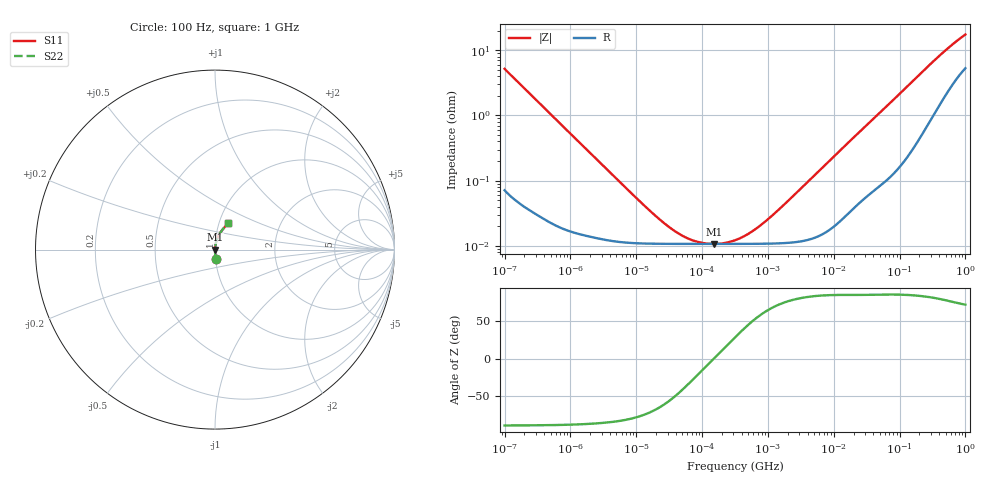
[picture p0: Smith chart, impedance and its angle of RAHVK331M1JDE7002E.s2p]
! RAHVK331M1JDE7002E  S-PARAMETER MODEL  (AEC-Q200 qualified)
! Model Generated by ELNA Corporation (http://www.ty-top.com)
! Version 1.0
! ELNA Control No.201026
! Copyright (c) 2020 ELNA CO.,LTD. All Rights Reserved.
! Products Name : CONDUCTIVE POLYMER HYBRID ALUMINUM ELECTROLYTIC CAPACITORS
! Characteristics :
!  Capacitance  :  330uF  ,  Rated voltage  :  6.3V
!  Operating Temp. Range  :  -55 to +125 degC  ,  Endurance  :  4000hr at 125 degC
!  Dimension D  :  6.3mm  ,  Dimension L  :  7.7mm
! Frequency Range : 100Hz - 1GHz
! External Node Assignments :
!  1  o---| |---o  2
# MHz S RI R 50
!Freq[MHz].  S11 Real  S11 Imag  S21 Real  S21 Imag  S12 Real  S12 Imag  S22 Real  S22 Imag
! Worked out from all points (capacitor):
!   401 points, 100 Hz to 1 GHz, reference 50 ohm
!   read as one part in series: C = 307 uF near 108 Hz
!   lowest |Z| = 10.7 mohm at 153.1 kHz (marker M1)
!   series resonance near 150.2 kHz, so ESL is about 3.7 nH
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0.0001  0.00338 -0.0515  0.9966 0.0515  0.9966 0.0515  0.00338 -0.0515
0.000113  0.00272 -0.0457  0.9973 0.0457  0.9973 0.0457  0.00272 -0.0457
0.000309  0.000582 -0.0168  0.9994 0.0168  0.9994 0.0168  0.000582 -0.0168
0.001488  0.00016 -0.00354  0.9998 0.00354  0.9998 0.00354  0.00016 -0.00354
0.009495  0.00011 -0.000559  0.9999 0.000559  0.9999 0.000559  0.00011 -0.000559
0.022131  0.000108 -0.000236  0.9999 0.000236  0.9999 0.000236  0.000108 -0.000236
0.037368  0.000107 -0.000134  0.9999 0.000134  0.9999 0.000134  0.000107 -0.000134
0.060604  0.000107 -7.38e-05  0.9999 7.38e-05  0.9999 7.38e-05  0.000107 -7.38e-05
0.094406  0.000107 -3.42e-05  0.9999 3.42e-05  0.9999 3.42e-05  0.000107 -3.42e-05
0.153109  0.000107 1.38e-06  0.9999 -1.38e-06  0.9999 -1.38e-06  0.000107 1.38e-06
0.220039  0.000107 2.78e-05  0.9999 -2.78e-05  0.9999 -2.78e-05  0.000107 2.78e-05
0.316228  0.000107 5.8e-05  0.9999 -5.8e-05  0.9999 -5.8e-05  0.000107 5.8e-05
0.512861  0.000107 0.000111  0.9999 -0.000111  0.9999 -0.000111  0.000107 0.000111
0.865964  0.000108 0.000199  0.9999 -0.000199  0.9999 -0.000199  0.000108 0.000199
1.650061  0.00011 0.000387  0.9999 -0.000387  0.9999 -0.000387  0.00011 0.000387
4.704354  0.00013 0.00111  0.9999 -0.00111  0.9999 -0.00111  0.00013 0.00111
69.9842  0.00133 0.0151  0.9987 -0.0151  0.9987 -0.0151  0.00133 0.0151
176.8072  0.00495 0.037  0.9951 -0.037  0.9951 -0.037  0.00495 0.037
395.8221  0.0197 0.0771  0.9803 -0.0771  0.9803 -0.0771  0.0197 0.0771
668.3439  0.0445 0.1147  0.9555 -0.1147  0.9555 -0.1147  0.0445 0.1147
922.5714  0.0671 0.1399  0.9329 -0.1399  0.9329 -0.1399  0.0671 0.1399
1000  0.0734 0.1463  0.9266 -0.1463  0.9266 -0.1463  0.0734 0.1463
